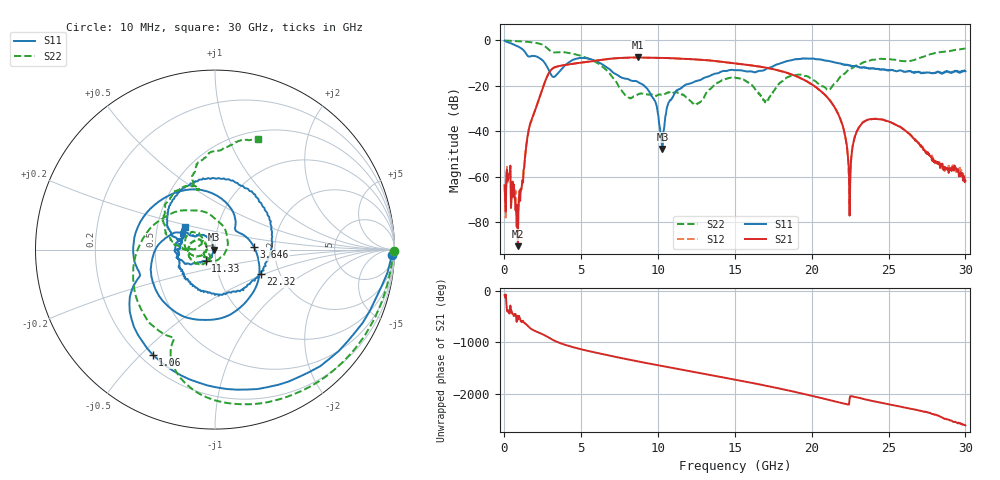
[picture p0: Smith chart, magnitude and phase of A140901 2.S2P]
!  2-Port S-parameters saved by WinCal
! VAR MeasName=S-Parameters (CALIBRATED_DATA) read from VNA (N5244A)
! VAR MeasDate=11/3/2014 9:26:40 AM
! VAR NAME=A140901 2
! VAR FILENAME=A140901 2.S2P
! VAR DATE=11/3/2014 9:26:40 AM
! VAR PHYS_PORTS=1,2
# Hz S RI R 50
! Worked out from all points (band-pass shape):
!   801 points, 10 MHz to 30 GHz, reference 50 ohm
!   highest |S21| = -7.53 dB at 8.67 GHz (marker M1); lowest = -90.6 dB at 872.2 MHz (marker M2)
!   |S21| within 3 dB of the highest: 4.191 GHz to 15.5 GHz (11.31 GHz wide, 115 % of centre)
!   lowest |S11| = -47.8 dB at 10.28 GHz (marker M3), VSWR 1.01, Z = 49.6 + j0.0442 ohm
!   |S11| at or under -10 dB: 2.63 GHz to 4.12 GHz (1.49 GHz wide, 44.2 % of centre); 6.231 GHz to 17.99 GHz (11.76 GHz wide, 97.1 % of centre); 21.68 GHz to end of sweep
!   |S22| runs from -28.3 to 0.0 dB; largest |S21 - S12| = 0.0036
!   S11 on the Smith chart (normalised r, x): 10 MHz: 24, -53; 1.06 GHz: 0.25, -0.54; 3.646 GHz: 1.56, +0.04; 11.33 GHz: 0.89, -0.12; 22.32 GHz: 1.60, -0.48; 30 GHz: 0.69, +0.19
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1e7  0.9855 -0.0307  0.000122 -0.000639  0.000622 -0.000213  0.9961 -0.00873
8.722125e8  -0.1405 -0.7237  -2.83e-05 8.87e-06  7.47e-06 7.08e-05  0.8119 -0.5102
1.05965e9  -0.3469 -0.5863  -0.000343 0.000424  -0.000388 0.000372  0.7397 -0.5984
1.734425e9  -0.4407 -0.0877  0.0158 -0.00434  0.0159 -0.00436  0.3866 -0.8253
2.484175e9  -0.1388 0.3353  -0.0453 -0.0762  -0.0453 -0.076  -0.1107 -0.7887
3.646288e9  0.2177 0.0135  0.1183 0.2499  0.1178 0.2497  -0.3008 -0.4598
5.033325e9  -0.2141 -0.3522  0.1809 -0.2698  0.1808 -0.2701  -0.4475 -0.0553
6.945188e9  -0.1941 0.0948  -0.396 0.0203  -0.3961 0.0205  0.00623 0.1669
8.669612e9  -0.0933 0.0794  0.1323 0.3989  0.1325 0.3984  -0.00773 -0.0634
1.001916e10  -0.0101 0.0194  0.4116 -0.0401  0.4107 -0.0399  -0.0479 -0.0424
1.028158e10  -0.00407 0.000445  0.3852 -0.1433  0.3848 -0.1426  -0.0468 -0.0421
1.133122e10  -0.0517 -0.0643  0.0741 -0.3909  0.0738 -0.3904  -0.0642 -0.0257
1.305565e10  -0.1294 -0.0812  -0.3688 -0.0295  -0.3685 -0.0279  -0.0298 -0.054
1.5005e10  -0.2213 0.0114  0.0789 0.3013  0.0807 0.2995  -0.1491 -0.00724
1.699184e10  -0.2203 0.0665  0.1915 -0.1634  0.1907 -0.164  -0.045 0.00714
2.002832e10  0.0776 0.3913  -0.0513 0.0932  -0.0518 0.0929  -0.0989 0.095
2.171526e10  0.3156 0.0156  0.0242 -0.0015  0.0242 -0.00135  -0.1345 0.00384
2.231506e10  0.2567 -0.1361  0.0028 -0.00272  0.00283 -0.00253  -0.2096 0.0233
2.25025e10  0.221 -0.1658  -0.000305 0.00069  -0.00046 0.0011  -0.2332 0.0295
2.332722e10  0.0392 -0.2532  0.00731 0.0138  0.00742 0.0141  -0.2865 0.1488
2.501416e10  -0.184 -0.113  0.0116 -0.0116  0.0117 -0.0116  -0.1607 0.3557
3e10  -0.1664 0.1274  -0.000101 -0.00082  0.000102 -0.000762  0.2378 0.6169
